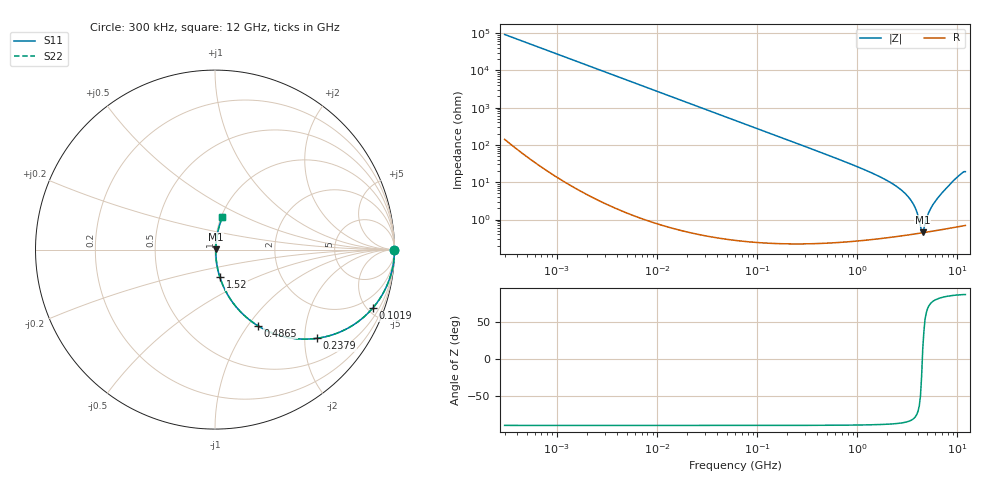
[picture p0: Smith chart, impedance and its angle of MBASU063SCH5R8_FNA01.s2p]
! MBASU063SCH5R8_FNA01  S-PARAMETER MODEL  ( General Type )
! Model Generated by TAIYO YUDEN Corporation (http://www.ty-top.com)
! Version 1.0
! TAIYO YUDEN Control No. 130801
! Copyright(c) 2013 TAIYO YUDEN CO.,LTD. All Rights Reserved.
! Product Description (link to TY-COMPAS)
! https://ds.yuden.co.jp/TYCOMPAS/or/detail?pn=MBASU063SCH5R8DFNA01&u=M
! Products Name : Multilayer Ceramic Capacitors
! Characteristics :
!  Capacitance : 5.8 pF , Rated Voltage : 50V , TCC : CH / C0H
!  Case Size : 0.6 x 0.3 / 0.024 x 0.012 [mm/inch] , Thickness : 0.3 / 0.012 [mm/inch]
!  (Conditions: Temperature = 25 degC , DC Bias Current/Voltage = 0A / 0V)
! External Node Assignments :
!  1  o---| |---o  2
! GND o---------o GND
! Frequency Range : 0.3MHz  -  12000MHz  [ 401 STEP ]
# MHz S RI R 50
! Freq[MHz].  S11 Real  S11 Imag  S21 Real  S21 Imag  S12 Real  S12 Imag  S22 Real  S22 Imag
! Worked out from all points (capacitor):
!   401 points, 300 kHz to 12 GHz, reference 50 ohm
!   read as one part in series: C = 5.8 pF near 316.3 kHz
!   lowest |Z| = 456 mohm at 4.503 GHz (marker M1)
!   series resonance near 4.458 GHz, so ESL is about 220 pH
!   S11 on the Smith chart (normalised r, x): 300 kHz: open; 101.9 MHz: 1.00, -5.38; 237.9 MHz: 1.00, -2.30; 486.5 MHz: 1.00, -1.11; 1.52 GHz: 1.01, -0.32; 12 GHz: 1.01, +0.38
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0.3  1 -0.00109  2.88e-06 0.00109  2.88e-06 0.00109  1 -0.00109
1.769972  1 -0.00645  4.39e-05 0.00645  4.39e-05 0.00645  1 -0.00645
10.44266  0.9985 -0.038  0.00146 0.038  0.00146 0.038  0.9985 -0.038
60  0.9542 -0.2087  0.0458 0.2087  0.0458 0.2087  0.9542 -0.2087
101.9188  0.8784 -0.3264  0.1216 0.3264  0.1216 0.3264  0.8784 -0.3264
237.9135  0.5691 -0.4942  0.4309 0.4942  0.4309 0.4942  0.5691 -0.4942
353.9943  0.3726 -0.482  0.6274 0.482  0.6274 0.482  0.3726 -0.482
486.4723  0.2378 -0.4237  0.7622 0.4237  0.7622 0.4237  0.2378 -0.4237
804.7407  0.0999 -0.296  0.9001 0.296  0.9001 0.296  0.0999 -0.296
1519.776  0.0275 -0.1546  0.9725 0.1546  0.9725 0.1546  0.0275 -0.1546
2088.533  0.0136 -0.1007  0.9864 0.1007  0.9864 0.1007  0.0136 -0.1007
2795.104  0.00713 -0.0588  0.9929 0.0588  0.9929 0.0588  0.00713 -0.0588
3364.605  0.00512 -0.0346  0.9949 0.0346  0.9949 0.0346  0.00512 -0.0346
3740.715  0.00454 -0.0214  0.9955 0.0214  0.9955 0.0214  0.00454 -0.0214
3944.255  0.00439 -0.0148  0.9956 0.0148  0.9956 0.0148  0.00439 -0.0148
4270.516  0.00433 -0.00509  0.9957 0.00509  0.9957 0.00509  0.00433 -0.00509
4502.883  0.0044 0.00113  0.9956 -0.00113  0.9956 -0.00113  0.0044 0.00113
4623.766  0.00446 0.00349  0.9955 -0.00349  0.9955 -0.00349  0.00446 0.00349
5278.635  0.00498 0.0166  0.995 -0.0166  0.995 -0.0166  0.00498 0.0166
6188.031  0.00619 0.0336  0.9938 -0.0336  0.9938 -0.0336  0.00619 0.0336
9207.246  0.0185 0.1103  0.9815 -0.1103  0.9815 -0.1103  0.0185 0.1103
12000  0.0417 0.1826  0.9583 -0.1826  0.9583 -0.1826  0.0417 0.1826
